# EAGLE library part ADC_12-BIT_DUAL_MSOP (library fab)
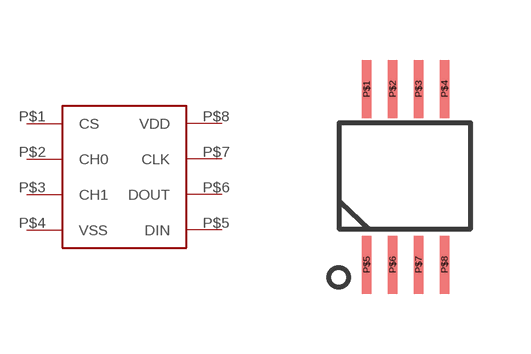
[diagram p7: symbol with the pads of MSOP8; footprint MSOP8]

Designator prefix -

## ADC_12-BIT_DUAL_MSOP  [MSOP8]
P$1  CS
P$2  CH0
P$3  CH1
P$4  VSS
P$5  DIN
P$6  DOUT
P$7  CLK
P$8  VDD

## Footprint MSOP8 (pad centres in mm)
smd 0.24 x 1.45: P$1 -0.65,2.45; P$2 0,2.45; P$3 0.65,2.45; P$4 1.3,2.45; P$5 -0.65,-1.95; P$6 0,-1.95; P$7 0.65,-1.95; P$8 1.3,-1.95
